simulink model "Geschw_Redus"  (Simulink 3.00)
settings: Solver=ode5  SolverMode=SingleTasking  StartTime=0.0  StopTime=0.4  RelTol=1e-3  AbsTol=1e-6
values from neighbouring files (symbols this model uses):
  alpha = 2*dR*TR*KI-(1/K_St)    [Red_Par.m]
  beta = 0    [Red_Par.m]
  bm = 4    [PI_Par.m]    (also in Red_Par.m)
  K_St = 1/FD_Stern    (= 2.27848101266)    [PI_Par.m]    (also in Red_Par.m = 1/FD_Stern)
  KI = T_St_max/(K_St*TR^2)    [Red_Par.m]
  qA = 0    [PI_Par.m]    (also in Red_Par.m)
  T_St = M_Stern/FD_Stern    (= 2.82860759494)    [PI_Par.m]    (also in Red_Par.m = M_Stern/FD_Stern)
  tb = vm/bm    (= 0.5)    [PI_Par.m]    (also in Red_Par.m)
  te = tv+tb    (= 1.2853981634)    [PI_Par.m]    (also in Red_Par.m)
  tv = se/vm    (= 0.785398163397)    [PI_Par.m]    (also in Red_Par.m)
  Vorz = 1    [PI_Par.m]    (also in Red_Par.m)
  z0 = (1/KM)*(rh)    (= 1.25)    [PI_Par.m]    (also in Red_Par.m = (1/KM)*(rh))

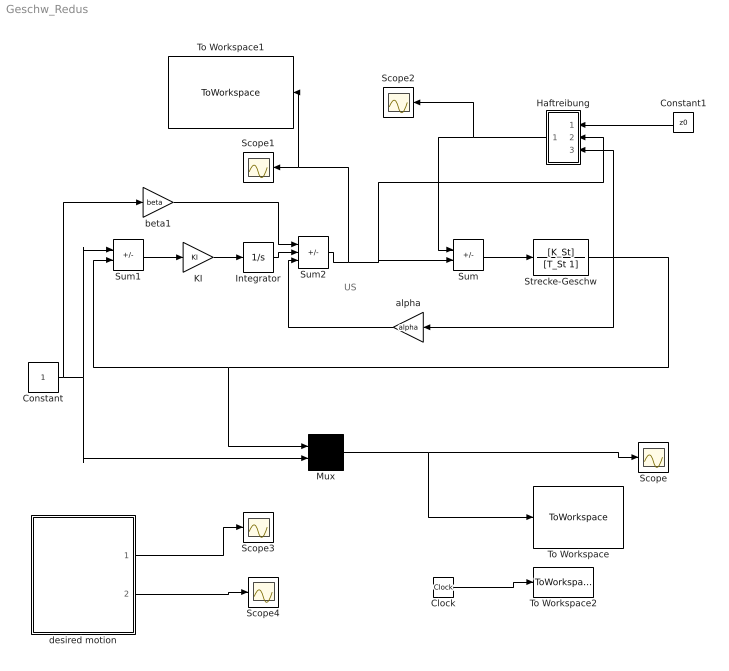
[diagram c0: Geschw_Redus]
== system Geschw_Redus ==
  note: US
  Clock : Clock
  Constant : Constant  Value=1
  Constant1 : Constant  Orientation=left  Value=z0
  Haftreibung : Subsystem  Orientation=left
  Integrator : Integrator  ExternalReset=none  InitialConditionSource=internal  InitialCondition=0  LimitOutput=off  UpperSaturationLimit=inf  LowerSaturationLimit=-inf  ShowSaturationPort=off  ShowStatePort=off  AbsoluteTolerance=auto
  KI : Gain  Gain=KI  SaturateOnIntegerOverflow=on
  Mux : Mux  Inputs=2
  Scope{,1..4} (5 alike) : Scope
  Strecke-Geschw : TransferFcn  Numerator=[K_St]  Denominator=[T_St 1]
  Sum : Sum  Inputs=-+  SaturateOnIntegerOverflow=on
  Sum1 : Sum  Inputs=+-  SaturateOnIntegerOverflow=on
  Sum2 : Sum  Inputs=++-  SaturateOnIntegerOverflow=on
  To Workspace : ToWorkspace  VariableName=Red_M_Min_SP  SampleTime=0.001  SaveFormat=Matrix
  To Workspace1 : ToWorkspace  VariableName=Red_M_Min_US_SP  SampleTime=0.001  SaveFormat=Matrix
  To Workspace2 : ToWorkspace  VariableName=Zeit_SP  SampleTime=0.001  SaveFormat=Matrix
  alpha : Gain  Orientation=left  Gain=alpha  SaturateOnIntegerOverflow=on
  beta1 : Gain  Gain=beta  SaturateOnIntegerOverflow=on
  desired motion : Subsystem
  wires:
  Strecke-Geschw/1 -> Sum1/2, Mux/1, Haftreibung/3(qp), alpha/1
  Sum/1 -> Strecke-Geschw/1
  Constant1/1 -> Haftreibung/1(z0)
  Haftreibung/1(Out1) -> Sum/1, Scope2/1
  Mux/1 -> Scope/1, To Workspace/1
  Clock/1 -> To Workspace2/1
  desired motion/1(qd) -> Scope3/1
  desired motion/2(vd) -> Scope4/1
  Sum1/1 -> KI/1
  KI/1 -> Integrator/1
  Sum2/1 -> Sum/2, Haftreibung/2(US), Scope1/1, To Workspace1/1
  Integrator/1 -> Sum2/2
  alpha/1 -> Sum2/3
  Constant/1 -> Mux/2, Sum1/1, beta1/1
  beta1/1 -> Sum2/1

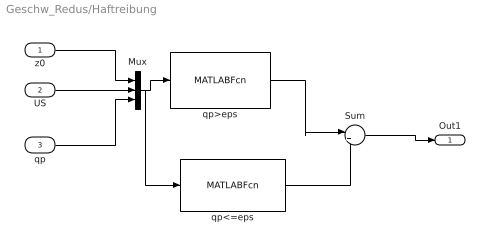
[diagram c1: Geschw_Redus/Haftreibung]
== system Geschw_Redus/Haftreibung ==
  z0 : Inport  Port=1  PortWidth=-1  SampleTime=-1  DataType=auto
  US : Inport  Port=2  PortWidth=-1  SampleTime=-1  DataType=auto
  qp : Inport  Port=3  PortWidth=-1  SampleTime=-1  DataType=auto
  Mux : Mux  Inputs=3
  Sum : Sum  Inputs=|++  SaturateOnIntegerOverflow=on
  qp<=eps : MATLABFcn  MATLABFcn=(abs(u(3)) < eps) *min(abs(u(2)),u(1))* sign(u(2))*sign(u(1))  OutputWidth=1  OutputSignalType=auto
  qp>eps : MATLABFcn  MATLABFcn=(abs(u(3)) > eps) * sign(u(3))*u(1)  OutputWidth=1  OutputSignalType=auto
  Out1 : Outport  Port=1  InitialOutput=0
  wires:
  z0/1 -> Mux/1
  US/1 -> Mux/2
  qp/1 -> Mux/3
  Mux/1 -> qp>eps/1, qp<=eps/1
  Sum/1 -> Out1/1
  qp>eps/1 -> Sum/1
  qp<=eps/1 -> Sum/2

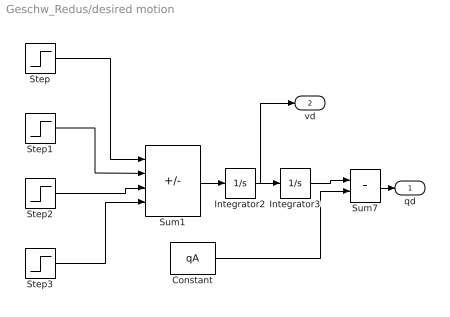
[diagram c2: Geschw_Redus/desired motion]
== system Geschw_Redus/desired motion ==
  Constant : Constant  Value=qA
  Integrator2 : Integrator  ExternalReset=none  InitialConditionSource=internal  InitialCondition=0  LimitOutput=off  UpperSaturationLimit=inf  LowerSaturationLimit=-inf  ShowSaturationPort=off  ShowStatePort=off  AbsoluteTolerance=auto
  Integrator3 : Integrator  ExternalReset=none  InitialConditionSource=internal  InitialCondition=0  LimitOutput=off  UpperSaturationLimit=inf  LowerSaturationLimit=-inf  ShowSaturationPort=off  ShowStatePort=off  AbsoluteTolerance=auto
  Step : Step  Time=0  Before=0  After=bm*Vorz  SampleTime=0.005
  Step1 : Step  Time=tb  Before=0  After=bm*Vorz  SampleTime=0.005
  Step2 : Step  Time=tv  Before=0  After=bm*Vorz  SampleTime=0.005
  Step3 : Step  Time=te  Before=0  After=bm*Vorz  SampleTime=0.005
  Sum1 : Sum  Inputs=+--+  SaturateOnIntegerOverflow=on
  Sum7 : Sum  Inputs=++  SaturateOnIntegerOverflow=on
  qd : Outport  Port=1  InitialOutput=0
  vd : Outport  Port=2
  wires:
  Step/1 -> Sum1/1
  Step1/1 -> Sum1/2
  Step2/1 -> Sum1/3
  Step3/1 -> Sum1/4
  Sum1/1 -> Integrator2/1
  Integrator2/1 -> Integrator3/1, vd/1
  Constant/1 -> Sum7/2
  Integrator3/1 -> Sum7/1
  Sum7/1 -> qd/1
